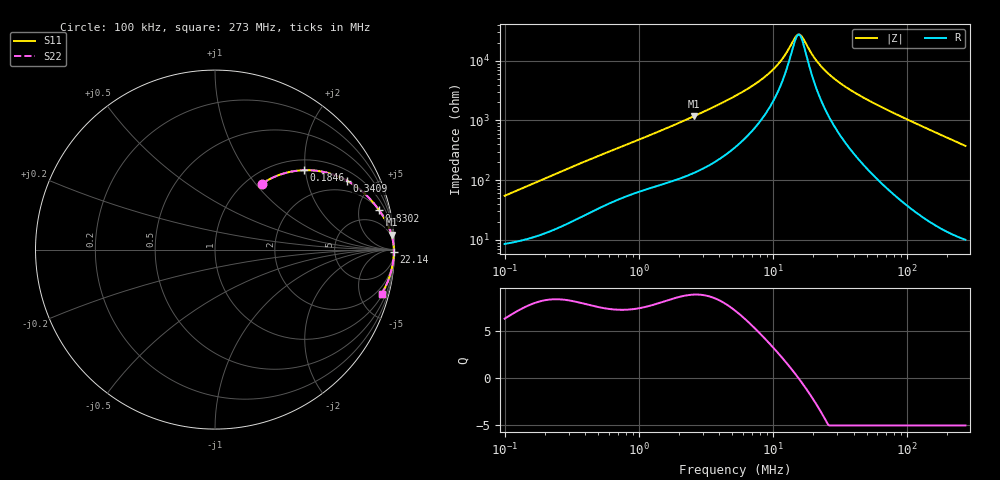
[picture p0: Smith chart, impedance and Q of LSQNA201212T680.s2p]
! LSQNA201212T680  S-PARAMETER MODEL  ( General Type )
! Model Generated by TAIYO YUDEN Corporation (http://www.ty-top.com)
! Version 2.0
! TAIYO YUDEN Control No. 100810NF25SB-FKC
! Copyright(c) 2007 TAIYO YUDEN CO.,LTD. All Rights Reserved.
! Product Description (link to TY-COMPAS)
! https://ds.yuden.co.jp/TYCOMPAS/or/detail?pn=LSQNA201212T680K&u=M
! Products Name : Inductors
! Characteristics :
!  Inductance : 68 uH , SRF(min) : 10 MHz , DC Resistance(max) : 7.8 Ohm
!  Rated Current : Saturation :70 mA , Temp Rise : 140 mA (40 degC)
!  Case Size : 2.0 x 1.25 / 0.079 x 0.049 [mm/inch] , Thickness : 1.25 / 0.049 [mm/inch]
!  (Conditions: Temperature = 25 degC , DC Bias Current/Voltage = 0A / 0V)
! External Node Assignments :
!  1  o---GGG---o  2
! GND o---------o GND
! Frequency Range : 0.1MHz  -  272.98108MHz  [ 402 STEP ]
# MHz S RI R 50
! Freq[MHz].  S11 Real  S11 Imag  S21 Real  S21 Imag  S12 Real  S12 Imag  S22 Real  S22 Imag
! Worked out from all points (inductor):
!   401 points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, 100 kHz to 273 MHz, reference 50 ohm
!   read as one part in series: L = 85.5 uH near 104 kHz
!   highest Q = 8.86 at 2.563 MHz (marker M1), where L = 72.2 uH
!   self-resonance near 15.51 MHz
!   S11 on the Smith chart (normalised r, x): 100 kHz: 1.17, +1.08; 184.6 kHz: 1.24, +1.97; 340.9 kHz: 1.44, +3.54; 830.2 kHz: 2.10, +7.96; 22.14 MHz: open; 273 MHz: 1.20, -7.50
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0.1  0.2614 0.3673  0.7386 -0.3673  0.7386 -0.3673  0.2614 0.3673
0.184629  0.496 0.4424  0.504 -0.4424  0.504 -0.4424  0.496 0.4424
0.340879  0.736 0.3834  0.264 -0.3834  0.264 -0.3834  0.736 0.3834
0.376316  0.766 0.3652  0.234 -0.3652  0.234 -0.3652  0.766 0.3652
0.830167  0.9152 0.2182  0.0848 -0.2182  0.0848 -0.2182  0.9152 0.2182
1.416134  0.9602 0.1426  0.0398 -0.1426  0.0398 -0.1426  0.9602 0.1426
2.563388  0.9836 0.0827  0.0164 -0.0827  0.0164 -0.0827  0.9836 0.0827
5.329134  0.9933 0.0373  0.0067 -0.0373  0.0067 -0.0373  0.9933 0.0373
7.608211  0.995 0.0227  0.00502 -0.0227  0.00502 -0.0227  0.995 0.0227
10.03569  0.9957 0.0133  0.00427 -0.0133  0.00427 -0.0133  0.9957 0.0133
11.99113  0.9961 0.0078  0.00393 -0.0078  0.00393 -0.0078  0.9961 0.0078
14.32759  0.9963 0.00248  0.00369 -0.00248  0.00369 -0.00248  0.9963 0.00248
15.20352  0.9964 0.000717  0.00363 -0.000717  0.00363 -0.000717  0.9964 0.000717
15.81703  0.9964 -0.000457  0.00359 0.000457  0.00359 0.000457  0.9964 -0.000457
16.45529  0.9964 -0.00163  0.00356 0.00163  0.00356 0.00163  0.9964 -0.00163
19.66158  0.9965 -0.00701  0.00346 0.00701  0.00346 0.00701  0.9965 -0.00701
22.13913  0.9966 -0.0107  0.00344 0.0107  0.00344 0.0107  0.9966 -0.0107
26.98136  0.9965 -0.0173  0.00352 0.0173  0.00352 0.0173  0.9965 -0.0173
34.20958  0.9962 -0.0262  0.00382 0.0262  0.00382 0.0262  0.9962 -0.0262
73.9896  0.9921 -0.0684  0.00791 0.0684  0.00791 0.0684  0.9921 -0.0684
144.9579  0.9769 -0.1365  0.0231 0.1365  0.0231 0.1365  0.9769 -0.1365
272.9811  0.9279 -0.2456  0.0721 0.2456  0.0721 0.2456  0.9279 -0.2456
